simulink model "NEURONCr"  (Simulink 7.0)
settings: Solver=ode45  StartTime=0.0  StopTime=tstop  RelTol=1e-3
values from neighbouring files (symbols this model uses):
  beta = 1    [ResCourV1.m]    (also in ResCrV1.m; ResEnerV1.m; Constantes.m = 0.95; ConstantesBck.m = 0.95)
  Cdl = 731.3E-9    (= 7.313e-07)    [ResCourV1.m]    (also in ResCrV1.m; ResEnerV1.m; Constantes.m = 6.03e-07; ConstantesBck.m = 6.03e-07)
  I0Stim = ResSinhCorr(iRes,2)*1E-3    [ResCrV1.m]    (also in ResEnerV1.m; WaveCompIET.m = 0; WaveCompIETIf.m = 0)
  Kf = 1    [ResCourV1.m]    (also in ResCrV1.m)
  Rct = 605.2E3    (= 605200)    [ResCourV1.m]    (also in ResCrV1.m; ResEnerV1.m; Constantes.m = 185600; ConstantesBck.m = 185600)
  sigma = 68000    [ResCourV1.m]    (also in ResCrV1.m; ResEnerV1.m; Constantes.m = 66466; ConstantesBck.m = 66466)
  T0Stim = ResSinhCorr(iRes,1)*1E-3    [ResCrV1.m]    (also in ResEnerV1.m; WaveCompIET.m = i; WaveCompIETIf.m = i)
  TypeStim = 11    [ResCrV1.m]    (also in ResEnerV1.m; WaveCompIET.m = 5; WaveCompIETIf.m = 5)
libraries: simulink x1

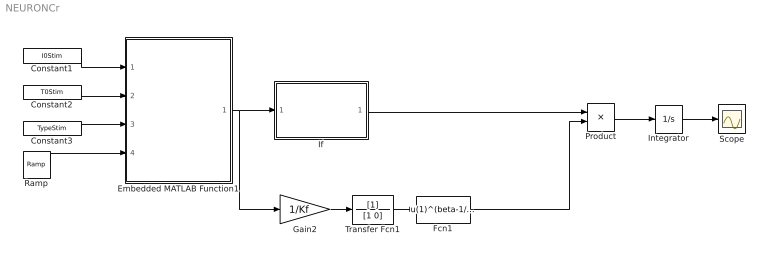
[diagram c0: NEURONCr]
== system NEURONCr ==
  Constant1 : Constant  Value=I0Stim  OutDataType=sfix(16)  OutScaling=2^0
  Constant2 : Constant  Value=T0Stim  OutDataType=sfix(16)  OutScaling=2^0
  Constant3 : Constant  Value=TypeStim  OutDataType=sfix(16)  OutScaling=2^0
  Embedded MATLAB Function1 : Stateflow chart
  Fcn1 : Fcn  Expr=u(1)^(beta-1/2)
  Gain2 : Gain  Gain=1/Kf  ParameterDataType=sfix(16)  ParameterScaling=2^0  OutDataType=sfix(16)  OutScaling=2^0
  If : Subsystem
  Integrator : Integrator
  Product : Product  OutDataType=sfix(16)  OutScaling=2^0
  Ramp : simulink/Sources/Ramp  SystemSampleTime=-1  slope=1  start=0  X0=0
  Scope : Scope
  Transfer Fcn1 : TransferFcn  Denominator=[1 0]
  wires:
  Constant1/1 -> Embedded MATLAB Function1/1(I0Stim)
  Constant2/1 -> Embedded MATLAB Function1/2(T0Stim)
  Constant3/1 -> Embedded MATLAB Function1/3(TypeStim)
  Ramp/1 -> Embedded MATLAB Function1/4(temps)
  Embedded MATLAB Function1/1(Istim) -> If/1(InZiet), Gain2/1
  If/1(OutZiet) -> Product/1
  Product/1 -> Integrator/1
  Integrator/1 -> Scope/1
  Transfer Fcn1/1 -> Fcn1/1
  Fcn1/1 -> Product/2
  Gain2/1 -> Transfer Fcn1/1

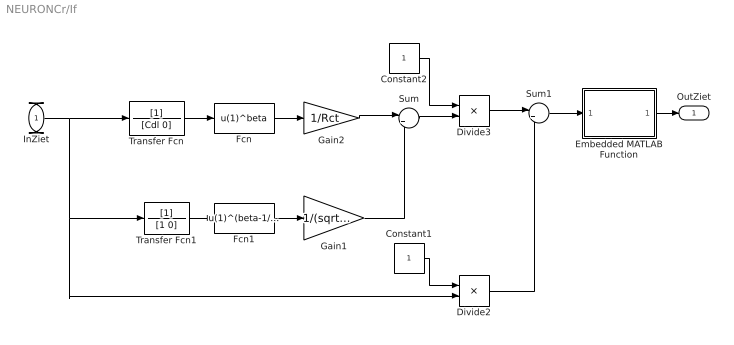
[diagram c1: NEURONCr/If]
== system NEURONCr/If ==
  InZiet : Inport  OutDataType=sfix(16)  OutScaling=2^0
  Constant1 : Constant  OutDataType=sfix(16)  OutScaling=2^0
  Constant2 : Constant  OutDataType=sfix(16)  OutScaling=2^0
  Divide2 : Product  Inputs=*/  OutDataType=sfix(16)  OutScaling=2^-10
  Divide3 : Product  Inputs=*/  OutDataType=sfix(16)  OutScaling=2^-10
  Embedded MATLAB Function : Stateflow chart
  Fcn : Fcn  Expr=u(1)^beta
  Fcn1 : Fcn  Expr=u(1)^(beta-1/2)
  Gain1 : Gain  Gain=1/(sqrt(2)*sigma*Cdl^beta)  ParameterDataType=sfix(16)  ParameterScaling=2^0  OutDataType=sfix(16)  OutScaling=2^0
  Gain2 : Gain  Gain=1/Rct  ParameterDataType=sfix(16)  ParameterScaling=2^0  OutDataType=sfix(16)  OutScaling=2^0
  Sum : Sum  Inputs=|++  OutDataType=sfix(16)  OutScaling=2^0
  Sum1 : Sum  Inputs=|++  OutDataType=sfix(16)  OutScaling=2^0
  Transfer Fcn : TransferFcn  Denominator=[Cdl 0]
  Transfer Fcn1 : TransferFcn  Denominator=[1 0]
  OutZiet : Outport  OutDataType=sfix(16)  OutScaling=2^0
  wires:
  Embedded MATLAB Function/1(y) -> OutZiet/1
  Transfer Fcn/1 -> Fcn/1
  InZiet/1 -> Transfer Fcn/1, Transfer Fcn1/1, Divide2/2
  Fcn/1 -> Gain2/1
  Transfer Fcn1/1 -> Fcn1/1
  Fcn1/1 -> Gain1/1
  Gain2/1 -> Sum/1
  Gain1/1 -> Sum/2
  Sum/1 -> Divide3/2
  Constant2/1 -> Divide3/1
  Constant1/1 -> Divide2/1
  Divide3/1 -> Sum1/1
  Divide2/1 -> Sum1/2
  Sum1/1 -> Embedded MATLAB Function/1(u)

== matlab function Embedded
MATLAB Function1 ==
function Istim = courant(I0Stim,T0Stim,TypeStim,temps)
% This block supports an embeddable subset of the MATLAB language.
% See the help menu for details. 

if temps <= T0Stim
    if TypeStim == 0
        Iout = I0Stim;
    elseif TypeStim == 1
        Iout = I0Stim*sin(pi/T0Stim*temps);
    elseif TypeStim == 2
        Iout = I0Stim*sin(pi/(2*T0Stim)*temps);
    elseif TypeStim == 3
        taum=0.07492974E-3;
        Iout = I0Stim*exp(temps/taum);
    elseif TypeStim == 4
        taum=0.07492974E-3;
        Iout = I0Stim*exp(-temps/taum);
    elseif TypeStim == 5
        Iout = I0Stim*(sin(pi/T0Stim*temps)+1/3*sin(3*pi/T0Stim*temps));
    elseif TypeStim == 6   
        taum=0.07492974E-3;
        Iout = I0Stim*sinh(temps/taum);
    elseif TypeStim == 7
        Iout = I0Stim*temps;
    elseif TypeStim == 8
        Iout = I0Stim*(T0Stim-temps);
    elseif TypeStim == 9
        Iout = I0Stim*(exp(-(5/sqrt(2))*((temps-T0Stim/2)/T0Stim)^2));
    elseif TypeStim == 10
        taum=0.2008E-3;
        Iout = I0Stim*exp(temps/taum);
    else
        taum = 4.07749143E-3;
        Iout = I0Stim*sinh(temps/taum);        
    end
else
    Iout = 0;
end
Istim = Iout;

== matlab function If/Embedded
MATLAB Function ==
function y = fcn(u)
% This block supports an embeddable subset of the MATLAB language.
% See the help menu for details. 

if u == Inf 
    y = 0;
else
    y = 1/u;
end
